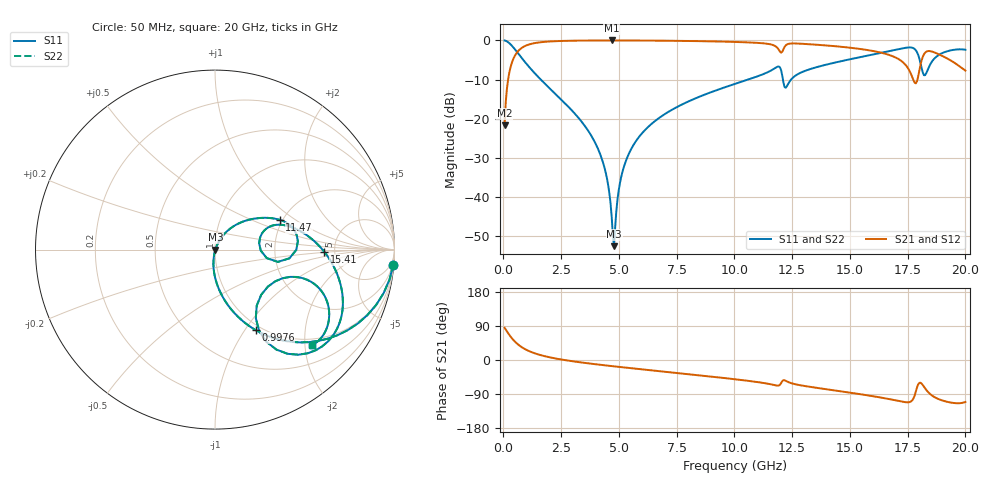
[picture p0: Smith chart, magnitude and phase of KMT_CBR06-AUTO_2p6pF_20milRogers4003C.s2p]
! Data measured by Modelithics Inc. support@modelithics.com 813-866-6335
! KEMET CBR06-AUTO 2.6pF, Pad Width= 0.851mm, Pad Length= 0.64mm, Pad Gap= 0.62mm, 20mil Rogers 4003C substrate Data, January 2022
# hz S ma R 50
! 2 Port Network Data from SP1.SP block
! freq  magS11  angS11  magS21  angS21  magS12  angS12  magS22  angS22
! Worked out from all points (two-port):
!   401 points, 50 MHz to 20 GHz, reference 50 ohm
!   highest |S21| = -0.02 dB at 4.688 GHz (marker M1); lowest = -21.7 dB at 50 MHz (marker M2)
!   |S21| within 3 dB of the highest: 595.2 MHz to 12 GHz (11.41 GHz wide, 181 % of centre); 12.05 GHz to 16.26 GHz (4.217 GHz wide, 29.8 % of centre)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
!   lowest |S11| = -52.5 dB at 4.788 GHz (marker M3), VSWR 1.00, Z = 50.2 - j0.0015 ohm
!   |S11| at or under -10 dB: 1.616 GHz to 10.59 GHz (8.974 GHz wide, 147 % of centre); 12.1 GHz to 12.46 GHz (355.2 MHz wide, 2.89 % of centre)
!   |S22| runs from -52.5 to 0.0 dB; largest |S21 - S12| = 0
!   S11 on the Smith chart (normalised r, x): 50 MHz: 1, -23; 997.6 MHz: 0.94, -1.12; 11.47 GHz: 1.93, +0.76; 15.41 GHz: 4.10, -0.15; 20 GHz: 0.85, -2.15
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5e7  0.9966 -4.9  0.0825 85.1  0.0825 85.1  0.9966 -4.9
3.4925e8  0.8642 -31.4  0.5021 58.6  0.5021 58.6  0.8642 -31.4
9.97625e8  0.5018 -63.2  0.8636 26.6  0.8636 26.6  0.5018 -63.2
3.391625e9  0.09124 -95.4  0.9938 -6.6  0.9938 -6.6  0.09124 -95.4
4.289375e9  0.02899 -99.1  0.9973 -13.3  0.9973 -13.3  0.02899 -99.1
4.53875e9  0.01398 -96.0  0.9975 -15.1  0.9975 -15.1  0.01398 -96.0
4.688375e9  0.005529 -82.1  0.9976 -16.1  0.9976 -16.1  0.005529 -82.1
4.788125e9  0.002374 -0.4  0.9976 -16.8  0.9976 -16.8  0.002374 -0.4
5.087375e9  0.01752 63.5  0.9973 -18.8  0.9973 -18.8  0.01752 63.5
5.386625e9  0.03357 65.1  0.9968 -20.7  0.9968 -20.7  0.03357 65.1
6.73325e9  0.1022 59.1  0.9917 -29.3  0.9917 -29.3  0.1022 59.1
1.0025e10  0.2787 38.2  0.9554 -50.8  0.9554 -50.8  0.2787 38.2
1.147138e10  0.3965 24.7  0.9007 -62.8  0.9007 -62.8  0.3965 24.7
1.192025e10  0.4641 5.8  0.7604 -67.3  0.7604 -67.3  0.4641 5.8
1.226938e10  0.2597 15.0  0.8856 -56.3  0.8856 -56.3  0.2597 15.0
1.336662e10  0.4383 17.0  0.888 -71.7  0.888 -71.7  0.4383 17.0
1.54115e10  0.6086 -1.1  0.7794 -89.8  0.7794 -89.8  0.6086 -1.1
1.670825e10  0.7288 -15.9  0.6507 -103.3  0.6507 -103.3  0.7288 -15.9
1.78055e10  0.7751 -48.2  0.2883 -93.4  0.2883 -93.4  0.7751 -48.2
1.810475e10  0.4441 -59.2  0.5556 -62.3  0.5556 -62.3  0.4441 -59.2
1.850375e10  0.5093 -18.1  0.7262 -91.4  0.7262 -91.4  0.5093 -18.1
2e10  0.7588 -44.8  0.4117 -110.8  0.4117 -110.8  0.7588 -44.8
